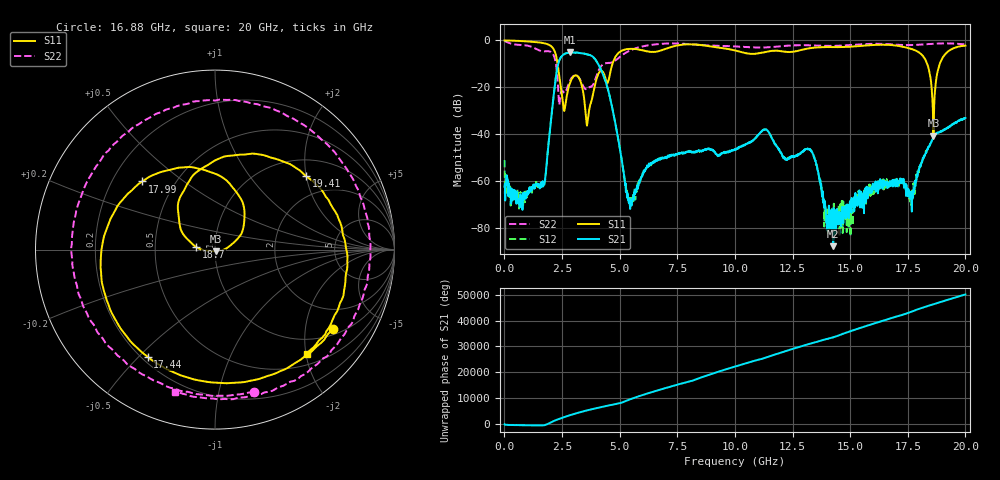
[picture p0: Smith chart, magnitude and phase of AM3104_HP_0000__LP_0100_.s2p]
!Created with skrf (http://scikit-rf.org).
# Hz S RI R 50.0
!freq ReS11 ImS11 ReS21 ImS21 ReS12 ImS12 ReS22 ImS22
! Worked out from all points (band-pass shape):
!   1601 points, 10 MHz to 20 GHz, reference 50 ohm
!   highest |S21| = -5.12 dB at 2.846 GHz (marker M1); lowest = -87.8 dB at 14.27 GHz (marker M2)
!   |S21| within 3 dB of the highest: 2.398 GHz to 3.945 GHz (1.546 GHz wide, 48.8 % of centre)
!   lowest |S11| = -40.6 dB at 18.61 GHz (marker M3), VSWR 1.02, Z = 50.3 - j0.877 ohm
!   |S11| at or under -10 dB: 2.308 GHz to 4.689 GHz (2.381 GHz wide, 68.1 % of centre); 18.34 GHz to 18.88 GHz (543.3 MHz wide, 2.92 % of centre)
!   |S22| runs from -27.4 to -0.2 dB; largest |S21 - S12| = 0.0043
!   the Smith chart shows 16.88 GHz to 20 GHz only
!   S11 on the Smith chart (normalised r, x): 16.88 GHz: 1.20, -2.81; 17.44 GHz: 0.22, -0.53; 17.99 GHz: 0.33, +0.36; 18.7 GHz: 0.81, +0.02; 19.41 GHz: 1.41, +2.00; 20 GHz: 0.69, -2.02
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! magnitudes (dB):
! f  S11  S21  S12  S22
! 10 MHz  0.0  -62.4  -51.1  -0.2
! 722.1 MHz  -0.2  -67.8  -67.5  -1.9
! 1.684 GHz  -1.1  -62.3  -61.0  -4.7
! 2.309 GHz  -10.0  -11.1  -11.1  -16.8
! 2.584 GHz  -29.8  -5.9  -5.9  -22.3
! 2.846 GHz  -18.2  -5.1  -5.1  -17.2
! 3.346 GHz  -18.8  -5.5  -5.5  -17.9
! 3.608 GHz  -34.5  -6.0  -6.0  -20.4
! 4.395 GHz  -16.4  -17.6  -17.6  -9.7
! 5.432 GHz  -3.5  -67.6  -69.1  -4.4
! 6.682 GHz  -4.6  -50.6  -50.9  -1.5
! 10.01 GHz  -4.2  -46.4  -46.6  -2.5
! 13.34 GHz  -3.1  -47.4  -47.8  -2.1
! 14.27 GHz  -2.8  -87.8  -74.6  -2.3
! 16.68 GHz  -1.9  -60.7  -61.6  -1.6
! 16.88 GHz  -2.1  -59.4  -61.9  -1.7
! 17.44 GHz  -3.0  -61.5  -61.9  -2.0
! 17.99 GHz  -5.1  -55.2  -55.6  -1.8
! 18.61 GHz  -40.6  -41.3  -41.2  -1.4
! 18.7 GHz  -19.4  -40.0  -39.9  -1.4
! 19.41 GHz  -3.7  -35.8  -35.7  -1.3
! 20 GHz  -2.2  -33.1  -33.1  -1.7
